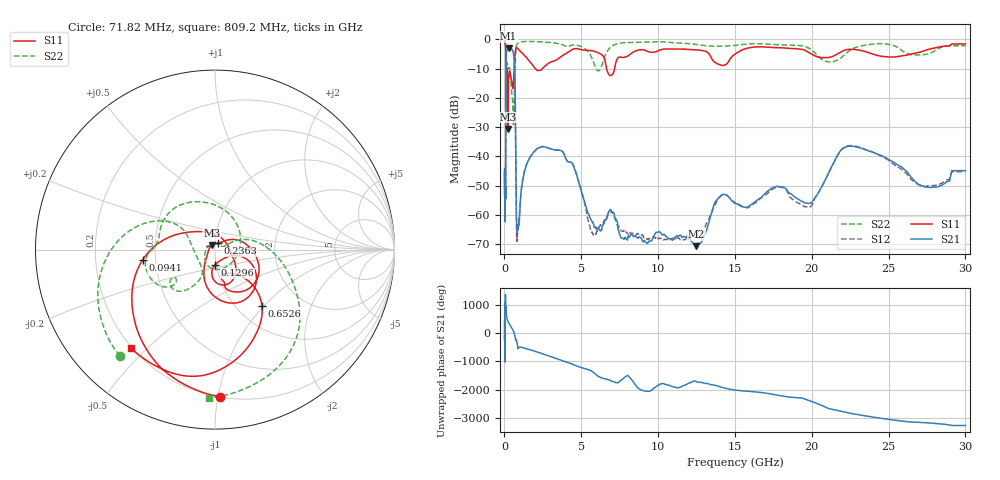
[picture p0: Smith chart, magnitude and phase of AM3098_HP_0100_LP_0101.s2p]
! Date/Time: Thu, Feb 28, 2019 8:35 AM
! Network Analyzer: Agilent Technologies E8364B Rev: A.07.50.67
! Sweep from 0.010 to 30.000 GHz, 1601 Points, Sweep Type: LOG
! Power Supply: 5.023 V, 0.002 A
# Hz S DB R 50
!freq MagS11 AngS11 MagS21 AngS21 MagS12 AngS12 MagS22 AngS22
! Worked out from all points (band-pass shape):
!   1601 points, 10 MHz to 30 GHz, reference 50 ohm
!   highest |S21| = -3.07 dB at 266.5 MHz (marker M1); lowest = -70.7 dB at 12.5 GHz (marker M2)
!   |S21| within 3 dB of the highest: 111.1 MHz to 618.6 MHz (507.5 MHz wide, 139 % of centre)
!   lowest |S11| = -30.6 dB at 229.3 MHz (marker M3), VSWR 1.06, Z = 48.2 + j2.28 ohm
!   |S11| at or under -10 dB: 176.7 MHz to 632.2 MHz (455.5 MHz wide, 113 % of centre); 2.022 GHz to 2.459 GHz (436.4 MHz wide, 19.5 % of centre); 6.647 GHz to 7.164 GHz (517.3 MHz wide, 7.49 % of centre)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
!   |S22| runs from -29.2 to -0.5 dB; largest |S21 - S12| = 0.011
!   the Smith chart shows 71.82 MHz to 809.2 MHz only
!   S11 on the Smith chart (normalised r, x): 71.82 MHz: 0.20, -1.01; 94.1 MHz: 0.42, -0.06; 129.6 MHz: 0.98, -0.17; 236.3 MHz: 1.03, +0.07; 652.6 MHz: 1.29, -0.98; 809.2 MHz: 0.19, -0.45
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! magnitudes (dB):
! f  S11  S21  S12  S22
! 10 MHz  -0.3  -45.9  -45.8  -0.5
! 38.04 MHz  -0.5  -61.9  -61.7  -0.9
! 71.82 MHz  -1.7  -52.6  -53.5  -2.0
! 94.1 MHz  -7.8  -20.9  -20.9  -9.3
! 129.6 MHz  -21.3  -4.3  -4.3  -10.8
! 144.7 MHz  -15.6  -3.8  -3.7  -10.7
! 184.9 MHz  -10.9  -3.6  -3.6  -8.0
! 229.3 MHz  -30.6  -3.2  -3.1  -9.6
! 236.3 MHz  -28.2  -3.1  -3.1  -9.7
! 266.5 MHz  -14.9  -3.1  -3.0  -9.9
! 550.5 MHz  -16.8  -4.1  -4.1  -24.8
! 652.6 MHz  -7.8  -8.7  -8.7  -17.5
! 809.2 MHz  -2.8  -65.0  -68.9  -1.6
! 2.084 GHz  -10.4  -37.5  -37.6  -0.7
! 3.76 GHz  -5.6  -38.3  -38.2  -1.7
! 5.725 GHz  -3.9  -62.6  -66.3  -6.8
! 7.926 GHz  -5.9  -68.3  -66.0  -1.1
! 12.5 GHz  -3.5  -70.7  -67.2  -1.7
! 14.16 GHz  -8.9  -53.1  -53.2  -2.3
! 19.7 GHz  -4.2  -56.0  -57.3  -2.7
! 22.56 GHz  -3.4  -36.5  -36.3  -3.5
! 30 GHz  -1.5  -44.9  -45.3  -2.2
